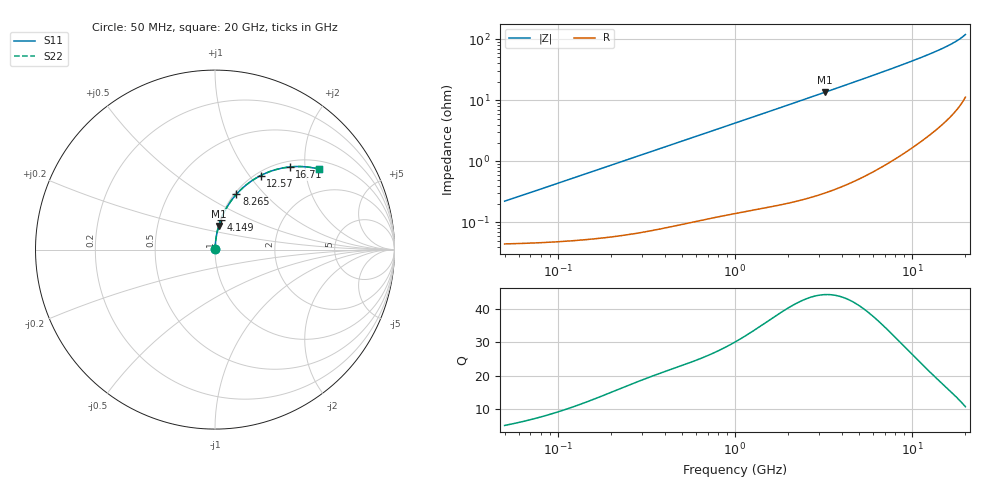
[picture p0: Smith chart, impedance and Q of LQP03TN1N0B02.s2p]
!Murata Part Number: LQP03TN1N0B02
!These Parameters are Measured in Series Mode Connection
!  o--[Z]--o
!Port1  Port2
!  o-------o
!Freq. Start=50[MHz] Stop=20[GHz], 401[Steps]
# Hz S RI R 50
!Freq.(Hz) S11(Real) S11(Imag) S21(Real) S21(Imag) S12(Real) S12(Imag) S22(Real) S22(Imag)
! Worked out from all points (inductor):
!   401 points, 50 MHz to 20 GHz, reference 50 ohm
!   read as one part in series: L = 695 pH near 51.52 MHz
!   highest Q = 44.5 at 3.217 GHz (marker M1), where L = 666 pH
!   S11 on the Smith chart (normalised r, x): 50 MHz: 1.00, +0.00; 4.149 GHz: 1.01, +0.35; 8.265 GHz: 1.02, +0.71; 12.57 GHz: 1.05, +1.14; 16.71 GHz: 1.11, +1.66; 20 GHz: 1.22, +2.36
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5e7  0.000451 0.00218  0.9995 -0.00218  0.9995 -0.00218  0.000451 0.00218
5.152053e7  0.000452 0.00225  0.9995 -0.00225  0.9995 -0.00225  0.000452 0.00225
5.895582e7  0.000458 0.00257  0.9995 -0.00257  0.9995 -0.00257  0.000458 0.00257
1.364002e8  0.000552 0.00592  0.9994 -0.00592  0.9994 -0.00592  0.000552 0.00592
3.721004e8  0.00103 0.0159  0.999 -0.0159  0.999 -0.0159  0.00103 0.0159
6.380365e8  0.00181 0.027  0.9982 -0.027  0.9982 -0.027  0.00181 0.027
1e9  0.00316 0.0419  0.9968 -0.0419  0.9968 -0.0419  0.00316 0.0419
1.714689e9  0.00697 0.0711  0.993 -0.0711  0.993 -0.0711  0.00697 0.0711
2.728004e9  0.0153 0.112  0.9847 -0.112  0.9847 -0.112  0.0153 0.112
3.216634e9  0.0206 0.1314  0.9794 -0.1314  0.9794 -0.1314  0.0206 0.1314
4.149438e9  0.033 0.1676  0.967 -0.1676  0.967 -0.1676  0.033 0.1676
5.683258e9  0.0596 0.2242  0.9404 -0.2242  0.9404 -0.2242  0.0596 0.2242
7.442007e9  0.0986 0.2835  0.9014 -0.2835  0.9014 -0.2835  0.0986 0.2835
8.264682e9  0.1198 0.3089  0.8802 -0.3089  0.8802 -0.3089  0.1198 0.3089
1.034674e10  0.1803 0.3654  0.8197 -0.3654  0.8197 -0.3654  0.1803 0.3654
1.149051e10  0.2173 0.3914  0.7827 -0.3914  0.7827 -0.3914  0.2173 0.3914
1.257102e10  0.2544 0.4125  0.7456 -0.4125  0.7456 -0.4125  0.2544 0.4125
1.460232e10  0.3295 0.4428  0.6705 -0.4428  0.6705 -0.4428  0.3295 0.4428
1.670968e10  0.4153 0.4603  0.5847 -0.4603  0.5847 -0.4603  0.4153 0.4603
1.828096e10  0.4866 0.4624  0.5134 -0.4624  0.5134 -0.4624  0.4866 0.4624
1.940974e10  0.5443 0.456  0.4557 -0.456  0.4557 -0.456  0.5443 0.456
2e10  0.5777 0.4488  0.4223 -0.4488  0.4223 -0.4488  0.5777 0.4488
